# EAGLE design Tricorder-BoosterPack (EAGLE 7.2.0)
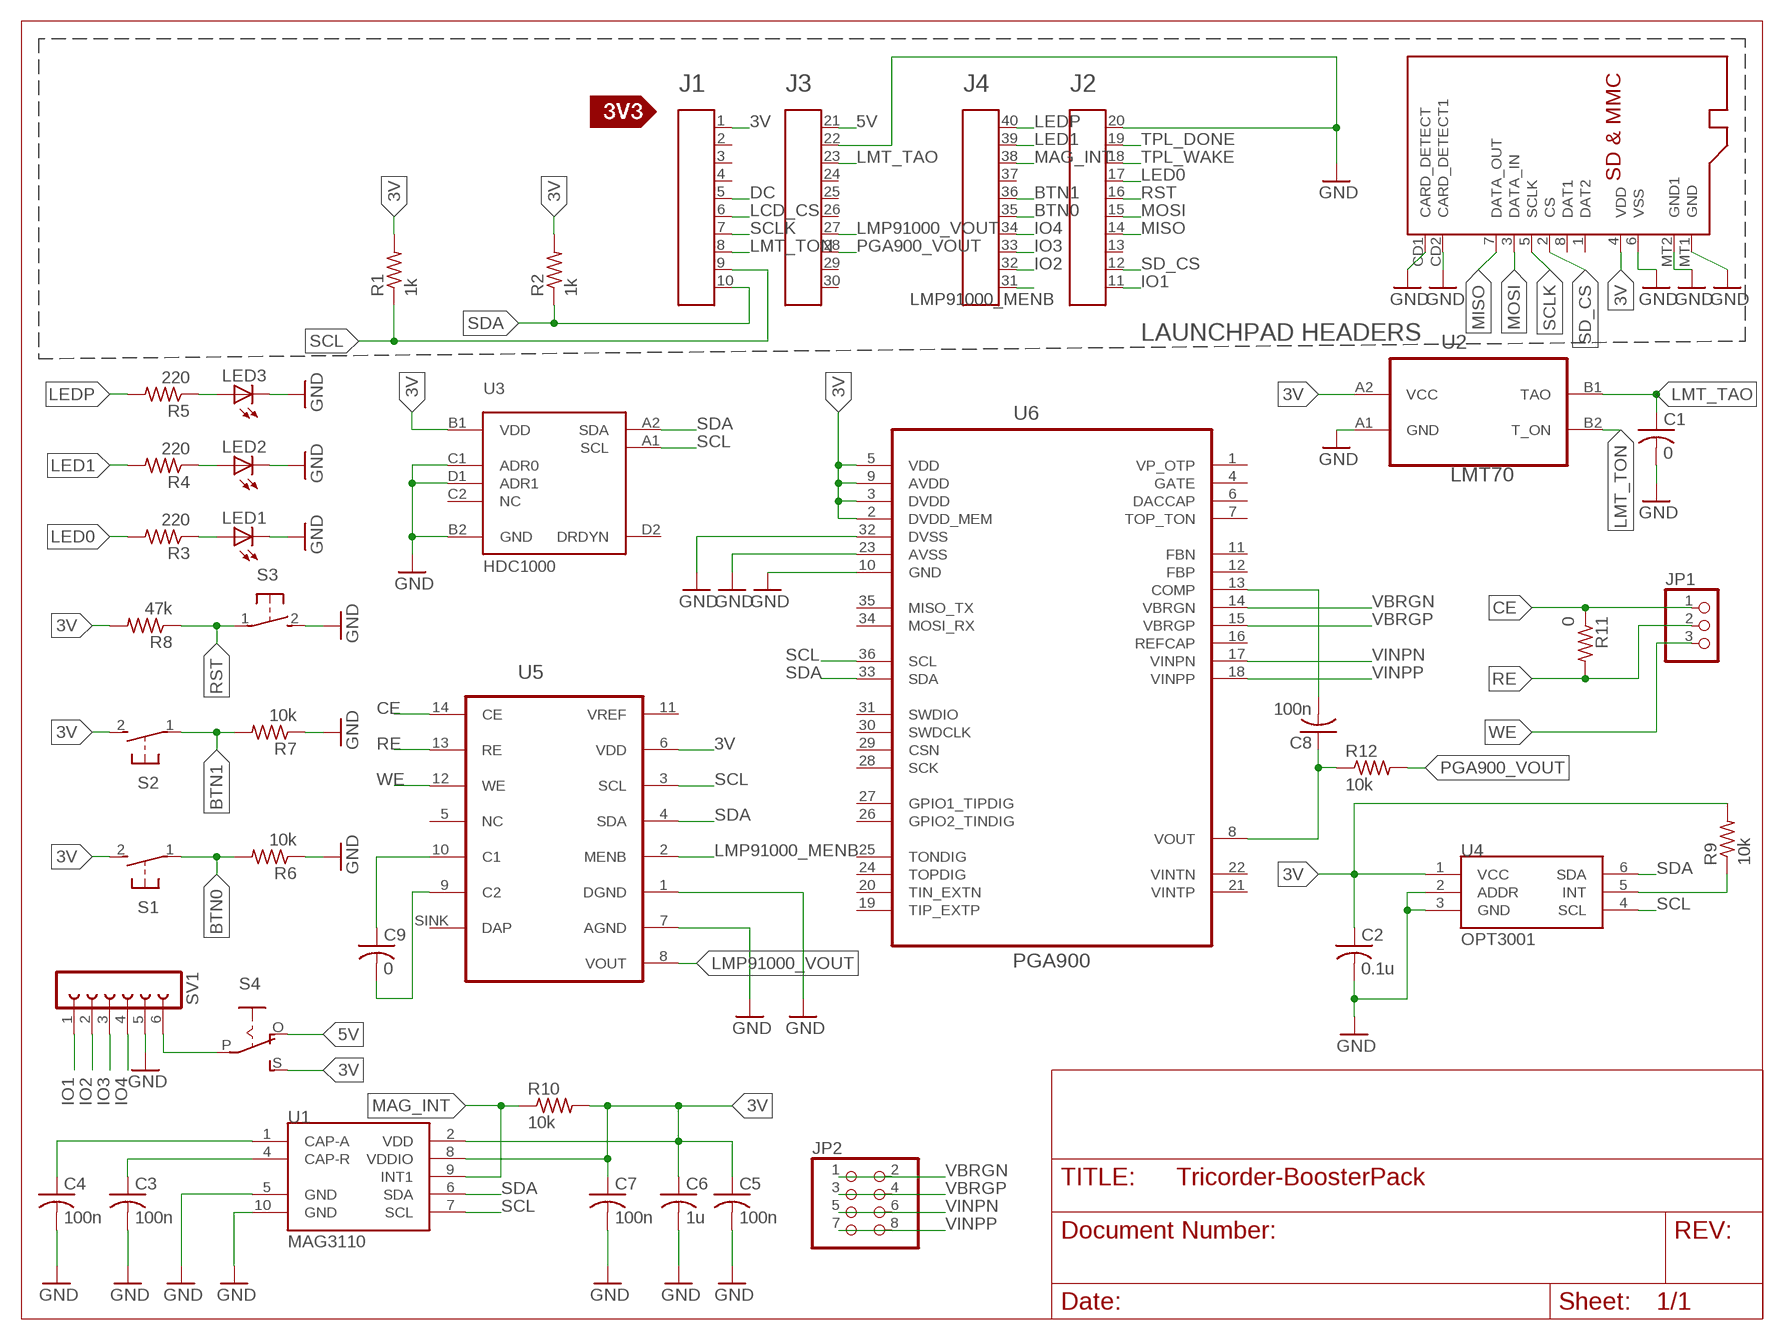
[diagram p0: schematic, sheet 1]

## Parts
A1  HEADER4X10-BOOSTERPACK  [4X10-BOOSTERPACK]
C1  0  C-USC0603  [C0603]
C2  0.1u  C-USC0603  [C0603]
C3  100n  C-USC0603  [C0603]
C4  100n  C-USC0603  [C0603]
C5  100n  C-USC0603  [C0603]
C6  1u  C-USC0603  [C0603]
C7  100n  C-USC0603  [C0603]
C8  100n  C-USC0603  [C0603]
C9  0  C-USC0603  [C0603]
JP1  PINHD-1X3CB  [1X03-CLEANBIG]
JP2  PINHD-2X4  [2X04]
LED1  LEDCHIPLED_0603  [CHIPLED_0603]
LED2  LEDCHIPLED_0603  [CHIPLED_0603]
LED3  LEDCHIPLED_0603  [CHIPLED_0603]
R1  1k  R-US_R0603  [R0603]
R2  1k  R-US_R0603  [R0603]
R3  220  R-US_R0603  [R0603]
R4  220  R-US_R0603  [R0603]
R5  220  R-US_R0603  [R0603]
R6  10k  R-US_R0603  [R0603]
R7  10k  R-US_R0603  [R0603]
R8  47k  R-US_R0603  [R0603]
R9  10k  R-US_R0603  [R0603]
R10  10k  R-US_R0603  [R0603]
R11  0  R-US_R0603  [R0603]
R12  10k  R-US_R0603  [R0603]
S1  31-XX  [B3F-31XX]
S2  31-XX  [B3F-31XX]
S3  31-XX  [B3F-31XX]
S4  EG1218S  [EG1218]
SV1  FE06-1  [FE06]
U1  MAG3110  [DFN-10]
U2  LMT70LMT70  [BGA4C40P2X2_77X77X50]
U3  HDC1000  [DSBGA_8_YPA]
U4  OPT3001  [SOT23-6]
U5  LMP91000  [WFDFN-14]
U6  PGA900  [QFN50P600X600X90-37N]
U7  MICROSD  [MICROSD]
U$3  SILK_3V3_TAG  [SILK_3V3_TAG]

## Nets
3V: A1.1 C2.1 R1.2 R2.2 R8.2 R9.2 S1.2(S) S2.2(S) S4.S U3.B1(VDD) U4.1(VCC) U5.6(VDD) U6.2(DVDD_MEM) U6.3(DVDD) U6.5(VDD) U6.9(AVDD) U7.4(VDD)
5V: A1.21 S4.O
BTN0: A1.35 R6.2 S1.1(P)
BTN1: A1.36 R7.2 S2.1(P)
CE: JP1.1 R11.1 U5.14(CE)
DC: A1.5
GND: A1.20 A1.22 C1.2 C2.2 C3.2 C4.2 C5.2 C6.2 C7.2 LED1.C LED2.C LED3.C R6.1 R7.1 S3.2(S) SV1.5 U1.5(GND) U1.10(GND) U2.A1(GND) U3.B2(GND) U3.C1(ADR0) U3.D1(ADR1) U4.2(ADDR) U4.3(GND) U5.1(DGND) U5.7(AGND) U6.10(GND) U6.23(AVSS) U6.32(DVSS) U7.6(VSS) U7.CD1(CARD_DETECT) U7.CD2(CARD_DETECT1) U7.MT1(GND) U7.MT2(GND1)
IO1: A1.11 SV1.1
IO2: A1.32 SV1.2
IO3: A1.33 SV1.3
IO4: A1.34 SV1.4
LCD_CS: A1.6
LED0: A1.17 R3.2
LED1: A1.39 R4.2
LEDP: A1.40 R5.2
LMP91000_MENB: A1.31 U5.2(MENB)
LMP91000_VOUT: A1.27 U5.8(VOUT)
LMT_TAO: A1.23 C1.1 U2.B1(TAO)
LMT_TON: A1.8 U2.B2(T_ON)
MAG_INT: A1.38 R10.1 U1.9(INT1)
MISO: A1.14 U7.7(DATA_OUT)
MOSI: A1.15 U7.3(DATA_IN)
N$1: LED1.A R3.1
N$2: LED2.A R4.1
N$3: LED3.A R5.1
N$4: S4.P SV1.6
N$5: R9.1 U4.5(INT)
N$6: U2.A2(VCC)
N$7: C9.1 U5.10(C1)
N$8: C3.1 U1.4(CAP-R)
N$9: C4.1 U1.1(CAP-A)
N$10: C8.2 U6.13(COMP)
N$11: C5.1 C6.1 C7.1 R10.2 U1.2(VDD) U1.8(VDDIO)
N$12: C8.1 R12.1 U6.8(VOUT)
N$13: C9.2 U5.9(C2)
PGA900_VOUT: A1.28 R12.2
RE: JP1.2 R11.2 U5.13(RE)
RST: A1.16 R8.1 S3.1(P)
SCL: A1.9 R1.1 U1.7(SCL) U3.A1(SCL) U4.4(SCL) U5.3(SCL) U6.36(SCL)
SCLK: A1.7 U7.5(SCLK)
SD_CS: A1.12 U7.2(CS)
SDA: A1.10 R2.1 U1.6(SDA) U3.A2(SDA) U4.6(SDA) U5.4(SDA) U6.33(SDA)
TPL_DONE: A1.19
TPL_WAKE: A1.18
VBRGN: JP2.1 JP2.2 U6.14(VBRGN)
VBRGP: JP2.3 JP2.4 U6.15(VBRGP)
VINPN: JP2.5 JP2.6 U6.17(VINPN)
VINPP: JP2.7 JP2.8 U6.18(VINPP)
WE: JP1.3 U5.12(WE)
Unconnected: A1.2 A1.3 A1.4 A1.13 A1.24 A1.25 A1.26 A1.29 A1.30 A1.37 U3.C2(NC) U3.D2(DRDYN) U5.5(NC) U5.SINK(DAP) U6.1(VP_OTP) U6.4(GATE) U6.6(DACCAP) U6.7(TOP_TON) U6.11(FBN) U6.12(FBP) U6.16(REFCAP) U6.19(TIP_EXTP) U6.20(TIN_EXTN) U6.21(VINTP) U6.22(VINTN) U6.24(TOPDIG) U6.25(TONDIG) U6.26(GPIO2_TINDIG) U6.27(GPIO1_TIPDIG) U6.28(SCK) U6.29(CSN) U6.30(SWDCLK) U6.31(SWDIO) U6.34(MOSI_RX) U6.35(MISO_TX) U7.1(DAT2) U7.8(DAT1)

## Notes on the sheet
- LAUNCHPAD HEADERS

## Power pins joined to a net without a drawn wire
VREF: U5.11(VREF)

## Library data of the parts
A1 = Public_BP_Library:HEADER4X10-BOOSTERPACK
C1-C9 = adafruit:C-US: CAPACITOR, American symbol
JP1 = adafruit:PINHD-1X3: PIN HEADER
JP2 = adafruit:PINHD-2X4: PIN HEADER
LED1-LED3 = adafruit:LED: LED
R1-R12 = resistor:R-US_: RESISTOR, American symbol
S1-S3 = adafruit:31-XX: OMRON SWITCH
S4 = adafruit:EG1218: SLIDING SWITCH 0.1" spacing through hole, vertical SPDT slide switch http://www.ladyada.net/library/pcb/eaglelibrary.html
SV1 = con-lsta:FE06-1: FEMALE HEADER; OC_FARNELL: unknown; OC_NEWARK: unknown
U1 = SparkFun-Sensors:MAG3110: 3-axis digital (I2C) magnetometer
U2 = LMT70:LMT70: LOW-POWER SINGLE INVERTER GATE; MPN: LMT70; OC_FARNELL: -; OC_NEWARK: 50R7866; PACKAGE: BGA-4; SUPPLIER: Texas Instruments
U3 = Fra:HDC1000
U4 = OPT3001:OPT3001
U5 = LMP91000:LMP91000: IC TI AFE for Gas Sensing; DIGIKEY: LMP91000SDE/NOPBCT-ND
U6 = PGA900:PGA900: Resistive Sensor Interface; MPN: PGA900; PACKAGE: QFN-36; SUPPLIER: TEXAS INSTRUMENTS
U7 = adafruit:MICROSD: Micro-SD / Transflash card holder with SPI pinout For the 3M # 2908-05WB-MG and/or 4UCON #19656 push-push type
U$3 = Public_BP_Library:SILK_3V3_TAG

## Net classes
0 default: width 0.15 mm, drill 0.508 mm, clearance 0.001 mm

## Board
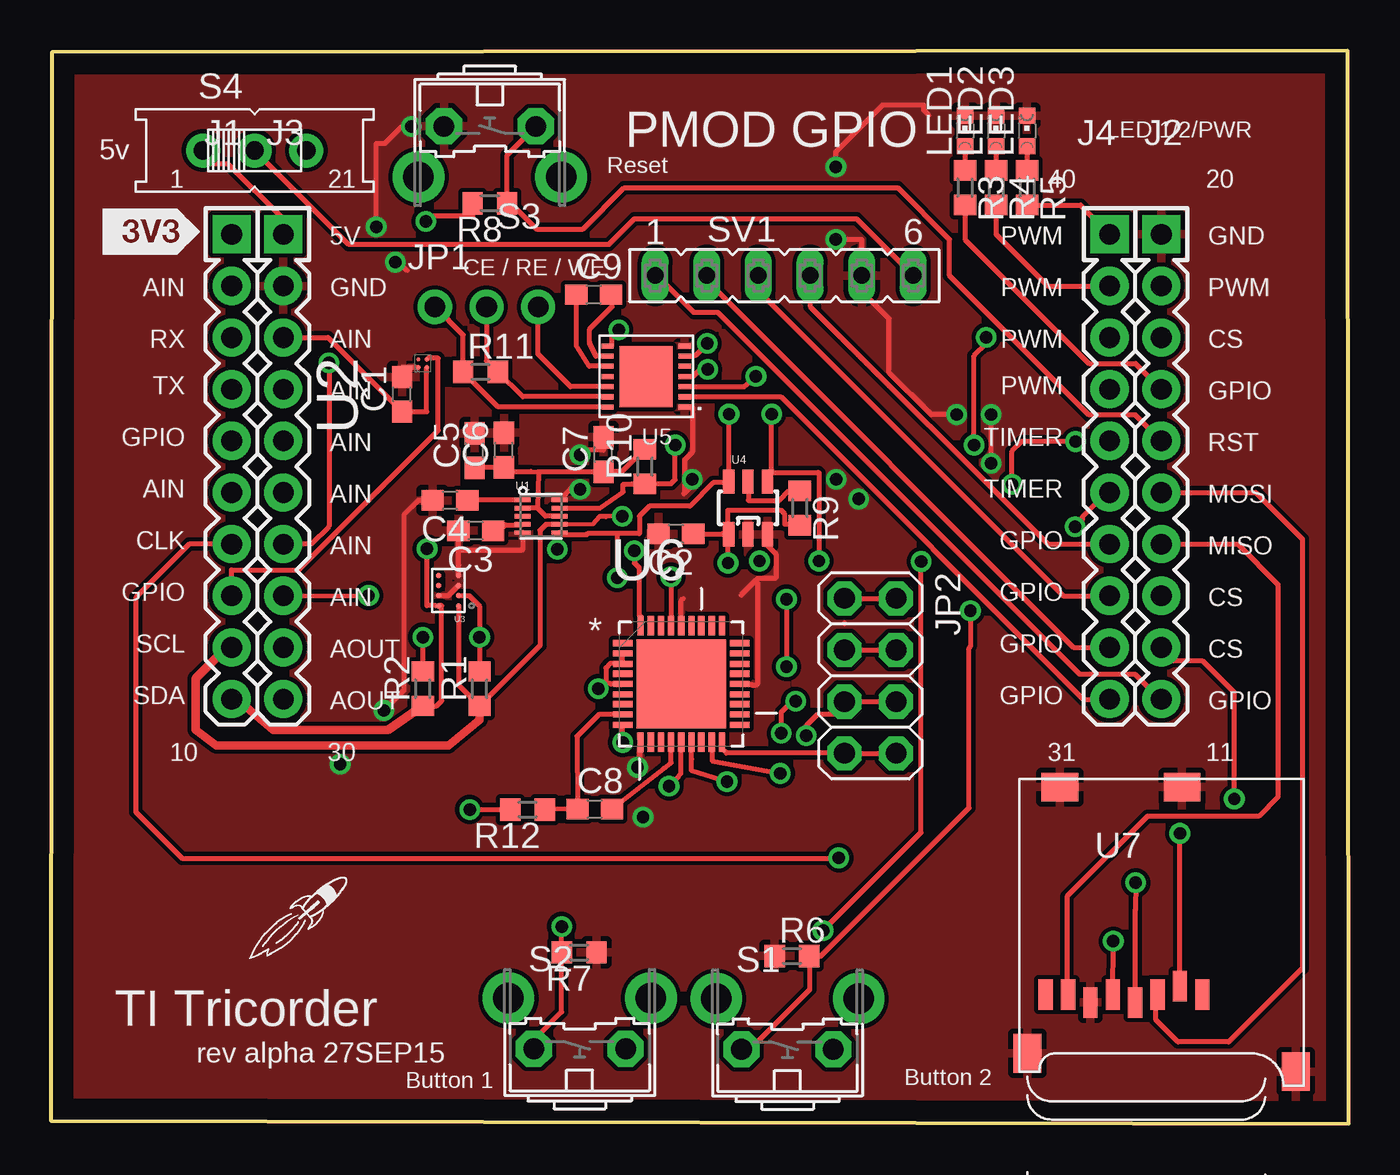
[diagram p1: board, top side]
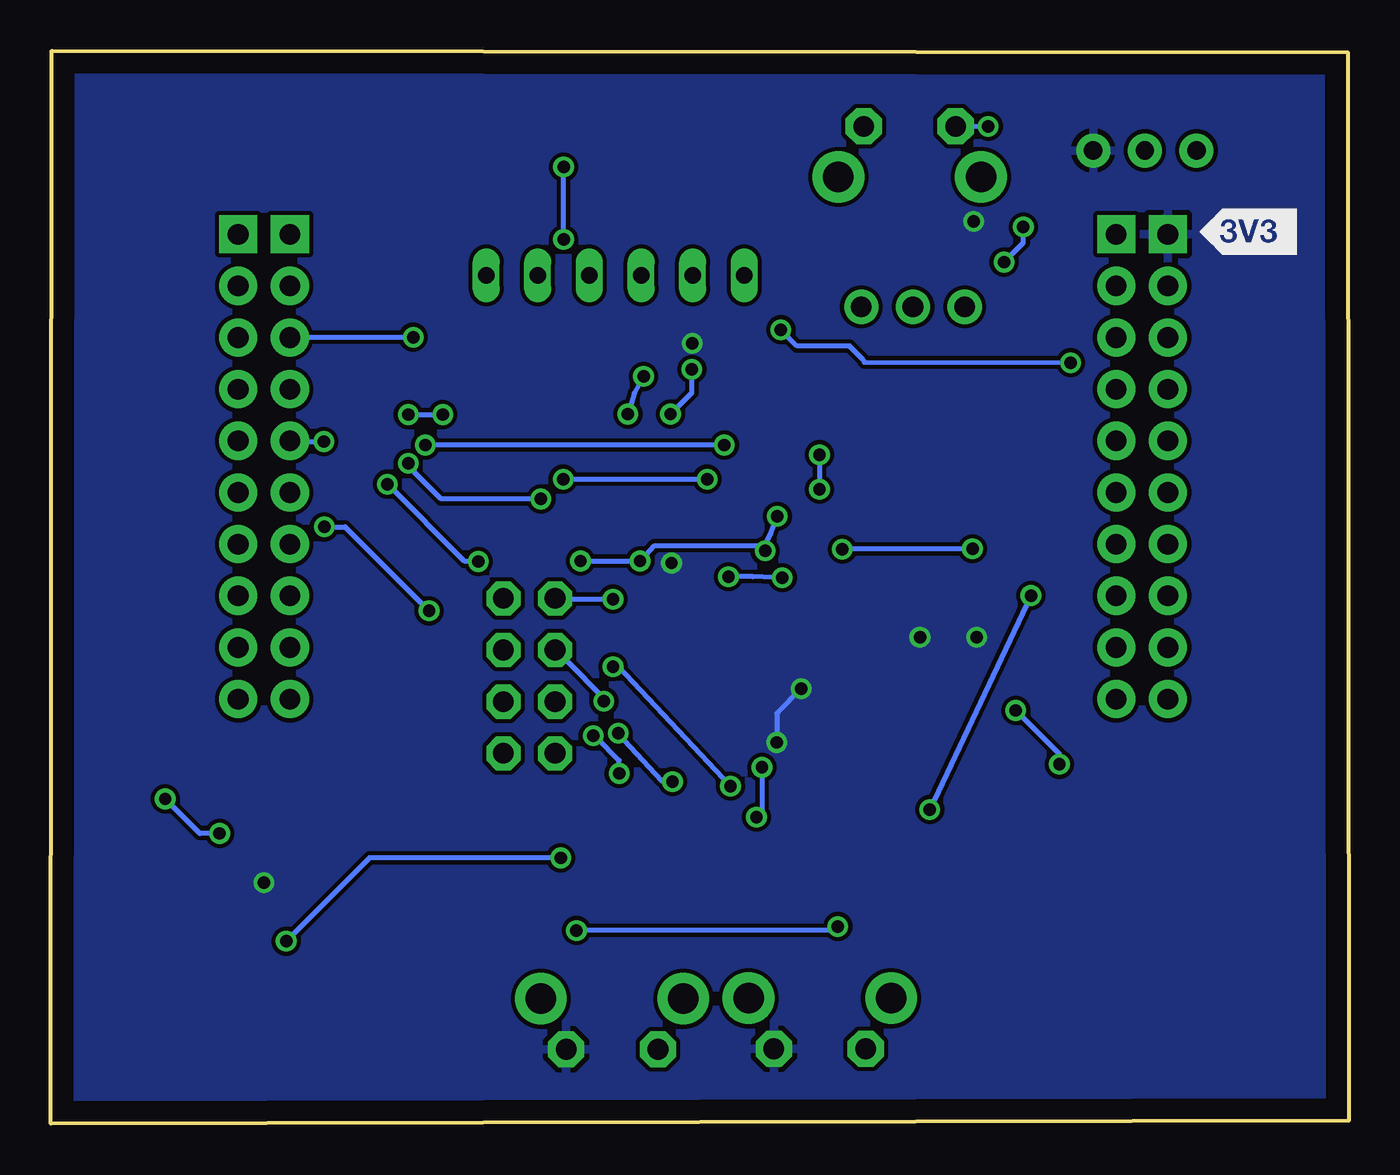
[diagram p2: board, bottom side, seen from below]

Size 63.82 x 52.77 mm. Coordinates in mm from the lower left corner, seen from the top.
Outline: 0,0.15 63.82,0 63.77,52.77 0.05,52.69 0,0.15
Copper layers (1*16): Top 0.035mm / dielectric 1.5mm / Bottom 0.035mm
Design rules "default": minimum track width 10mil, minimum drill 24mil, track to track 8mil, track to pad 8mil, pad to pad 8mil, via to via 8mil, smd to smd 8mil, copper to edge 40mil, drill to drill 8mil, minimum pad ring 10mil, minimum via ring 8mil, stop-mask expansion 4mil, vias tented up to drill 0mil, thermal gap 10mil

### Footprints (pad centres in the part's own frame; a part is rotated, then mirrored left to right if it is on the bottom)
4X10-BOOSTERPACK = drill 1.016 pad 1.88 square: 1 0,10.16; 20 45.72,10.16; 21 2.54,10.16; 40 43.18,10.16 | drill 1.016 pad 1.88: 2 0,7.62; 3 0,5.08; 4 0,2.54; 5 0,0; 6 0,-2.54; 7 0,-5.08; 8 0,-7.62; 9 0,-10.16; 10 0,-12.7; 11 45.72,-12.7; 12 45.72,-10.16; 13 45.72,-7.62; 14 45.72,-5.08; 15 45.72,-2.54; 16 45.72,0; 17 45.72,2.54; 18 45.72,5.08; 19 45.72,7.62; 22 2.54,7.62; 23 2.54,5.08; 24 2.54,2.54; 25 2.54,0; 26 2.54,-2.54; 27 2.54,-5.08; 28 2.54,-7.62; 29 2.54,-10.16; 30 2.54,-12.7; 31 43.18,-12.7; 32 43.18,-10.16; 33 43.18,-7.62; 34 43.18,-5.08; 35 43.18,-2.54; 36 43.18,0; 37 43.18,2.54; 38 43.18,5.08; 39 43.18,7.62
C0603 = smd 1.1 x 1: 1 -0.85,0; 2 0.85,0
1X03-CLEANBIG = drill 1.016 pad 1.676: 1 -2.54,0; 2 0,0; 3 2.54,0
2X04 = drill 1.016 pad 1.676 octagon: 1 -3.81,-1.27; 2 -3.81,1.27; 3 -1.27,-1.27; 4 -1.27,1.27; 5 1.27,-1.27; 6 1.27,1.27; 7 3.81,-1.27; 8 3.81,1.27
CHIPLED_0603 = smd 0.8 x 0.8: A 0,-0.75; C 0,0.75
R0603 = smd 1 x 1.1: 1 -0.85,0; 2 0.85,0
B3F-31XX = drill 1.016 pad 1.778 octagon: 1 -2.261,-1.245; 2 2.261,-1.245 | drill 1.499 pad 2.54: 3 -3.505,1.245; 4 3.505,1.245
EG1218 = drill 0.9 pad 1.676: O -2.54,0; P 0,0; S 2.54,0
FE06 = drill 0.813 long: 1 -6.35,0; 2 -3.81,0; 3 -1.27,0; 4 1.27,0; 5 3.81,0; 6 6.35,0
DFN-10 = smd 0.8 x 0.22: 1 -0.91,0.8; 2 -0.91,0.4; 3 -0.91,0; 4 -0.91,-0.4; 5 -0.91,-0.8; 6 0.91,-0.8; 7 0.91,-0.4; 8 0.91,0; 9 0.91,0.4; 10 0.91,0.8
BGA4C40P2X2_77X77X50 = smd 0.203 x 0.203: A1 -0.203,0.203; A2 0.203,0.203; B1 -0.203,-0.203; B2 0.203,-0.203
DSBGA_8_YPA = smd 0.275 x 0.275: A1 -0.5,0.75; A2 0.5,0.75; B1 -0.5,0.25; B2 0.5,0.25; C1 -0.5,-0.25; C2 0.5,-0.25; D1 -0.5,-0.75; D2 0.5,-0.75
SOT23-6 = smd 0.55 x 1.2: 1 -0.95,-1.3; 2 0,-1.3; 3 0.95,-1.3; 4 0.95,1.3; 5 0,1.3; 6 -0.95,1.3
WFDFN-14 = smd 0.25 x 0.6: 1 -1.5,-1.9; 2 -1,-1.9; 3 -0.5,-1.9; 4 0,-1.9; 5 0.5,-1.9; 6 1,-1.9; 7 1.5,-1.9; 8 1.5,1.9; 9 1,1.9; 10 0.5,1.9; 11 0,1.9; 12 -0.5,1.9; 13 -1,1.9; 14 -1.5,1.9 | smd 3 x 2.6: SINK 0,0
QFN50P600X600X90-37N = smd 0.965 x 0.305: 1 -2.87,2.007; 2 -2.87,1.499; 3 -2.87,0.991; 4 -2.87,0.508; 5 -2.87,0; 6 -2.87,-0.508; 7 -2.87,-0.991; 8 -2.87,-1.499; 9 -2.87,-2.007; 19 2.87,-2.007; 20 2.87,-1.499; 21 2.87,-0.991; 22 2.87,-0.508; 23 2.87,0; 24 2.87,0.508; 25 2.87,0.991; 26 2.87,1.499; 27 2.87,2.007 | smd 0.305 x 0.965: 10 -2.007,-2.87; 11 -1.499,-2.87; 12 -0.991,-2.87; 13 -0.508,-2.87; 14 0,-2.87; 15 0.508,-2.87; 16 0.991,-2.87; 17 1.499,-2.87; 18 2.007,-2.87; 28 2.007,2.87; 29 1.499,2.87; 30 0.991,2.87; 31 0.508,2.87; 32 0,2.87; 33 -0.508,2.87; 34 -0.991,2.87; 35 -1.499,2.87; 36 -2.007,2.87 | smd 4.394 x 4.394: 37 0,0
MICROSD = smd 0.7 x 1.5: 1 9,-10.64; 2 7.9,-10.24; 3 6.8,-10.64; 4 5.7,-11.04; 5 4.6,-10.64; 6 3.5,-11.04; 7 2.4,-10.64; 8 1.3,-10.64 | smd 1.8 x 1.4: CD1 2,-0.44; CD2 8,-0.44 | smd 1.4 x 1.9: MT1 0.4,-13.54; MT2 13.6,-14.44

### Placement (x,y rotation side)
A1  8.89,33.59 0 top
C1  17.27,35.87 90 top
C2  30.73,29.01 180 top
C3  20.9,29.16 180 top
C4  19.62,30.65 180 top
C5  20.84,33.1 90 top
C6  22.28,33.14 90 top
C7  27.18,32.91 90 top
C8  26.75,15.47 0 top
C9  26.7,40.77 0 top
JP1  21.42,40.18 0 top
JP2  40.3,22.03 270 top
LED1  44.96,48.83 0 top
LED2  46.48,48.83 0 top
LED3  48.01,48.83 0 top
R1  21.08,21.39 90 top
R2  18.29,21.39 90 top
R3  44.96,46.03 270 top
R4  46.48,46.03 270 top
R5  48.01,46.03 270 top
R6  36.45,8.25 0 top
R7  25.98,8.42 180 top
R8  21.59,45.27 180 top
R9  36.83,30.28 270 top
R10  29.21,32.32 90 top
R11  21.12,36.98 0 top
R12  23.45,15.45 180 top
S1  36.22,4.91 0 top
S2  26.01,4.93 0 top
S3  21.59,47.81 180 top
S4  10.02,47.86 0 top
SV1  36.07,41.71 0 top
U1  24.11,29.88 0 top
U2  18.29,37.4 90 top
U3  19.56,26.22 180 top
U4  34.29,30.28 0 top
U5  29.27,36.75 90 top
U6  31,21.62 0 top
U7  47.62,17 0 top
U$2  [LOGO-ROCKET]  12.32,10.31 0 top
U$3  2.54,42.73 0 top

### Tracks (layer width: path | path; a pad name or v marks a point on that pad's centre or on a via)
3V  (via drill 0.61)
  Top 0.254: 21.08,22.16 R1.2 v21.08,23.93 21.08,25.46 20.57,25.97 U3.B1 | v18.29,23.93 R2.2 | 20.83,45.27 R8.2 20.75,45.15 20.75,44.62 18.72,44.62 18.45,44.35 v18.45,44.38 | 33.02,29.01 U4.1 | 36.83,29.52 R9.2 36.8,29.48 36.1,29.48 36.1,29.98 35.9,30.18 33.3,30.18 33.3,29.08 U4.1 | C2.1 33.31,29.01 U4.1 | v33.3,27.58 33.3,28.88 U4.1 | U5.6 31.57,37.75 31.62,37.8 31.73,37.8 32.27,38.35 v32.27,38.38 | U6.2 28.12,23.1 U6.3 28,22.62 27.5,22.62 27.3,22.43 27.3,21.7 | 27.3,21.7 27.32,21.68 27.47,21.68 27.52,21.62 U6.5 | v28.12,18.75 28.12,19.6 U6.9 | v26.92,21.4 27.17,21.65 27.3,21.7 | U7.4 53.32,10.5 v53.35,11.85
  Bottom 0.254: v28.12,18.75 28.12,20.2 v26.92,21.4
  pour Bottom: -0.63,53.77 -0.63,0.01 64.24,-0.01 64.31,53.75
5V
  Top 0.254: A1.21 11.43,43.88 11.43,44.5 8.7,47.23 7.47,47.23 S4.O
BTN0  (via drill 0.61)
  Top 0.254: 52.07,31.03 A1.35 51.95,31.05 50.73,29.83 50.73,29.7 v50.38,29.35 | S1.1 34.39,3.66 37.32,6.6 37.32,8.22 R6.2 37.88,8.25 45.15,15.53 45.15,23.38 45.17,23.4 45.23,23.53 v45.23,25.23
  Bottom 0.254: v45.23,25.23 49.35,29.35 v50.38,29.35
BTN1  (via drill 0.61)
  Top 0.254: S2.1 23.75,4.32 23.95,4.32 25.12,5.5 R7.2 25.12,8.55 v25.12,9.7 | v50.4,33.55 47.75,33.55 47.27,33.08 v47.27,31.45 | v42.8,27.65 42.8,14.32 v37.98,9.5
  Bottom 0.254: v50.4,33.55 51.17,33.55 51.2,33.58 52.05,33.58 A1.36 | v47.27,31.45 43.48,27.65 v42.8,27.65 | v37.98,9.5 25.32,9.5 v25.12,9.7
CE
  Top 0.254: U5.14 22,35.25 R11.1 20.27,38.79 JP1.1
GND  (via drill 0.61)
  Top 0.254: 17.53,41.97 17.03,42.46 | 17.03,42.46 16.76,42.73 | 43.18,49.59 42.93,49.84 42.93,50.09 40.89,50.09 38.61,47.81 v38.61,47.05 | v38.61,43.49 39.88,43.49 SV1.5 39.88,41.6 39.88,40.95 41.23,39.6 41.23,36.95 43.3,34.88 v44.55,34.88 | U2.A1 17.27,37.19 C1.2 | 29.95,28.98 C2.2 | v17.72,49.05 17.27,49.05 16.42,48.2 16,48.2 v16,44.1 | v16.95,42.38 17.03,42.46 | 34.66,26.71 34.77,26.83 35.65,26.83 35.65,28.03 35.25,28.43 U4.3 | 34.66,26.71 33.95,26 | U6.32 31,25.73 31.1,25.83 | U6.23 34.2,21.62 34.23,21.6 34.5,21.6 34.52,21.58 34.67,21.58 34.7,21.6 34.75,21.6 34.75,26.62 34.66,26.71 | v28.85,17.53 28.95,17.62 28.95,18.25 29,18.3 U6.10 | 31.17,31.03 31.55,31.4 v31.55,31.7 | 31.17,31.03 31.12,30.98 | 31.17,31.03 31.17,32.65 31.55,33.02 31.55,35.23 31.52,35.25 U5.1 | 39.05,24.65 39.05,24.59 | v46.25,32.48 v46.25,34.88 | U3.D1 20.06,27.47 20.05,28.22 | 20.05,28.22 C3.2 | U3.B2 19.56,25.97 U3.C1 | v26.02,31.2 25.92,31.2 25.8,31.33 25.67,31.33 U1.10 | v26.02,32.9 26.25,33.12 27.17,33.12 C7.2 | v14.22,17.68 14.22,17.5 | v16.38,20.33 17.35,21.3 17.35,29.93 18.07,30.65 18.75,30.65 C4.2 | U1.5 23.2,28.25 23.15,28.2 20.08,28.2 20.05,28.22
  Bottom 0.254: v38.61,43.49 v38.61,47.05 | v17.72,49.05 S3.2 | v16,44.1 16,43.33 v16.95,42.38 | v29.12,15.07 29.1,15.07 28.85,15.32 v28.85,17.53 | v38.62,31.7 v31.55,31.7 | v46.25,34.88 v44.55,34.88 | v46.25,32.48 45.95,32.18 45.95,32.05 44.62,30.73 v39.73,30.73 | v26.02,32.9 v26.02,31.2 | v14.22,17.68 14.22,18.18 v16.38,20.33
  pour Top: -0.58,53.75 -0.58,0.06 64.29,0.14 64.26,53.67
IO1
  Top 0.254: A1.11 54.54,20.89 53.32,22.1 50.6,22.1 32.8,39.9 31.62,39.9 29.81,41.71 SV1.1
IO2
  Top 0.254: SV1.2 32.26,41.46 50.29,23.43 A1.32
IO3
  Top 0.254: SV1.3 34.8,40.95 49.78,25.96 A1.33
IO4
  Top 0.254: SV1.4 37.34,40.19 49.02,28.51 A1.34
LED0
  Top 0.254: R3.2 44.96,43.49 51.05,37.4 53.34,37.4 A1.17
LED1
  Top 0.254: R4.2 46.48,43.75 49.02,41.2 A1.39
LEDP
  Top 0.254: R5.2 50.63,45.18 A1.40
LMP91000_MENB
  Top 0.254: U5.2 35.9,35.75 50.77,20.88 52.06,20.88 A1.31
LMP91000_VOUT  (via drill 0.61)
  Top 0.254: v13.68,37.43 13.68,29.38 12.8,28.5 A1.27 | U5.8 27.57,38.25 27.57,38.7 v27.92,39.05
  Bottom 0.254: v13.68,37.43 23.82,37.45 23.88,37.58 24.55,38.25 27.12,38.25 v27.92,39.05
LMT_TAO
  Top 0.254: U2.B1 18.49,35.02 C1.1 13.63,38.66 A1.23
LMT_TON
  Top 0.254: A1.8 8.89,27.24 12.19,27.24 19.05,34.09 19.05,37.65 18.54,37.65 U2.B2
MAG_INT  (via drill 0.61)
  Top 0.254: v45.4,33.38 45.4,37.77 46,38.38 v46,38.68 | v30.7,33.38 30.7,31.68 30.5,31.48 29.3,31.48 R10.1 28.56,31.46 28.15,31.45 28.15,31.08 27,30.28 U1.9
  Bottom 0.254: v30.7,33.38 v45.4,33.38 | v46,38.68 52,38.68 A1.38
MISO
  Top 0.254: A1.14 58.37,28.51 60.35,26.53 60.35,16.08 59.4,15.12 53.92,15.12 49.98,11.17 49.98,6.41 U7.7
MOSI
  Top 0.254: A1.15 59.25,31.05 61.55,28.75 61.55,7.65 57.92,4.02 55.42,4.02 54.35,5.1 54.35,6.28 U7.3
N$1
  Top 0.254: LED1.A R3.1
N$2
  Top 0.254: LED2.A R4.1
N$3
  Top 0.254: LED3.A R5.1
N$4
  Top 0.254: SV1.6 39.62,44.51 28.7,44.51 27.43,43.24 14.65,43.24 S4.P
N$5
  Top 0.254: 34.3,31.68 U4.5 34.3,30.65 35.82,30.65 36.31,31.13 R9.1 36.9,31.08 37,31.18 36.9,31.28
N$7
  Top 0.254: U5.10 26.47,37.25 25.85,38.25 C9.1
N$8
  Top 0.254: C3.1 22.3,29.4 22.35,29.45 23.17,29.45 U1.4
N$9
  Top 0.254: U1.1 20.5,30.68 C4.1
N$10
  Top 0.254: C8.2 30.15,17.48 30.5,17.75 U6.13
N$11
  Top 0.254: R10.2 28.09,32.07 C7.1 26.72,32.05 23.97,32.05 | C5.1 20.88,32.29 C6.1 22.49,32.08 23.6,32.08 23.97,32.05 | U1.8 24.32,29.88 23.92,30.28 | 23.92,30.28 U1.2 | 23.97,32.05 23.92,30.28
N$12
  Top 0.254: U6.8 26.95,20.13 25.88,19.05 C8.1 R12.1
N$13
  Top 0.254: U5.9 26.8,37.75 26.5,38.43 26.5,39.08 27.6,40.18 27.6,40.73 C9.2 27.45,40.68
PGA900_VOUT  (via drill 0.61)
  Top 0.254: v20.6,15.45 R12.2 | A1.28 v15.63,25.98
  Bottom 0.254: v15.63,25.98 v20.6,15.45
RE
  Top 0.254: JP1.2 21.42,37.52 R11.2 23.2,35.75 U5.13
RST
  Top 0.254: S3.1 22.44,47.64 R8.1 22.61,45.27 23.88,44 26.16,44 28.19,46.03 41.66,46.03 44.2,43.49 44.2,41.71 51.05,34.86 53.34,34.86 A1.16
SCL  (via drill 0.61)
  Top 0.22: 26.97,29.85 26.67,29.5 U1.7
  Top 0.254: A1.9 8.64,23.43 | U3.A1 20.06,21.57 R1.1 24.05,23.51 24.05,29.18 24.35,29.48 U1.7 | v37.77,27.68 37.77,32 37.75,32.02 35.25,32.02 35.25,31.6 U4.4 35.45,32.15 v35.45,34.9 35.45,35.2 | 26.97,29.85 27.3,29.85 v28.1,29.88 | v34.67,36.75 34.1,36.25 U5.3 | U6.36 29,24.95 28.95,25 28.95,27.33 28.7,27.58 v28.7,28.18
  Top 0.406: 8.64,23.43 7.11,21.9 7.11,19.36 8.13,18.6 19.56,18.6 21.08,19.87 R1.1
  Bottom 0.254: v37.77,27.68 v34.85,27.68 34.73,27.78 34.12,28.43 28.7,28.43 | v28.1,29.88 28.42,29 28.7,28.43 | v35.45,34.9 35.12,35.95 v34.67,36.75 | v28.7,28.18 28.7,28.43
SCLK  (via drill 0.61)
  Top 0.254: U7.5 v52.25,8.97 | A1.7 6.8,28.51 4.18,25.88 4.18,15.32 6.45,13.05 38.73,13.05 v38.75,13.07
  Bottom 0.254: v38.75,13.07 48.15,13.07 v52.25,8.97
SD_CS  (via drill 0.61)
  Top 0.254: A1.12 54.6,23.43 54.6,22.78 56.62,22.78 58.2,21.2 v58.2,15.97 | U7.2 v55.52,14.28
  Bottom 0.254: v58.2,15.97 56.5,14.28 v55.52,14.28
SDA  (via drill 0.61)
  Top 0.254: A1.10 9.14,20.89 | R2.1 18.5,20.58 18.5,20.55 18.97,20.55 19.22,20.8 19.22,25.48 19.07,25.48 U3.A2 18.92,25.48 18.5,25.48 v18.5,28.28 | v24.9,28.25 24.9,29 U1.6 25.12,29 25.12,28.98 26.35,28.98 26.4,29.03 27.85,29.03 | U5.4 31.57,36.75 31.82,37 32.17,37 32.3,37.12 v32.3,37.1 | v33.35,34.9 33.35,31.6 U4.6 33.23,31.53 32.57,31.53 31.42,30.38 29.45,30.38 28.95,29.88 28.95,29.03 27.85,29.03 | v30.5,26.9 U6.33 | 27.85,29.03 v27.85,26.85
  Top 0.406: 9.14,20.89 10.92,19.36 16.6,19.36 R2.1
  Bottom 0.254: v24.9,28.25 24.88,28.28 v18.5,28.28 | v32.3,37.1 32.3,35.95 v33.35,34.9 | v30.5,26.9 29.3,26.9 v27.85,26.85
VBRGN  (via drill 0.61)
  Top 0.254: JP2.1 JP2.2 | U6.14 31,18.55 30.98,18.53 30.98,17.23 30.85,17.05 v30.4,16.6 | v36.17,25.8 v36.17,22.48
  Bottom 0.254: v30.4,16.6 35.92,22.48 v36.17,22.48 | v36.17,25.8 38.3,25.8 38.32,25.83 JP2.1
VBRGP  (via drill 0.61)
  Top 0.254: JP2.3 JP2.4 | v35.92,19.2 35.92,20.25 36.62,20.95 v36.62,20.78 | v33.25,16.83 31.5,17.38 31.51,17.93 U6.15
  Bottom 0.254: v36.62,20.78 36.62,20.93 38.5,22.8 38.5,23.3 JP2.3 | v33.25,16.83 33.77,16.85 v35.92,19.2
VINPN  (via drill 0.61)
  Top 0.254: JP2.6 JP2.5 39.02,20.65 39.02,20.12 37.7,20.12 37.15,19.58 v37.15,19.08 | v35.88,17.23 32.52,17.85 32.52,18.75 U6.17
  Bottom 0.254: v37.15,19.08 37.05,18.98 36.98,18.98 35.88,17.88 v35.88,17.23
VINPP
  Top 0.254: JP2.8 JP2.7 33.23,18.23 33.01,18.44 U6.18
WE
  Top 0.254: U5.12 25.55,36.25 23.95,37.85 23.95,40.16 JP1.3

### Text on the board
tPlace: PMOD GPIO | LED 1/2/PWR | 5v | Reset | CE / RE / WE | TI Tricorder | rev alpha 27SEP15 | Button 1 | Button 2

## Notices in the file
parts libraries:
SparkFun-Sensors: Licensing: Creative Commons ShareAlike 4.0 International - https://creativecommons.org/licenses/by-sa/4.0
